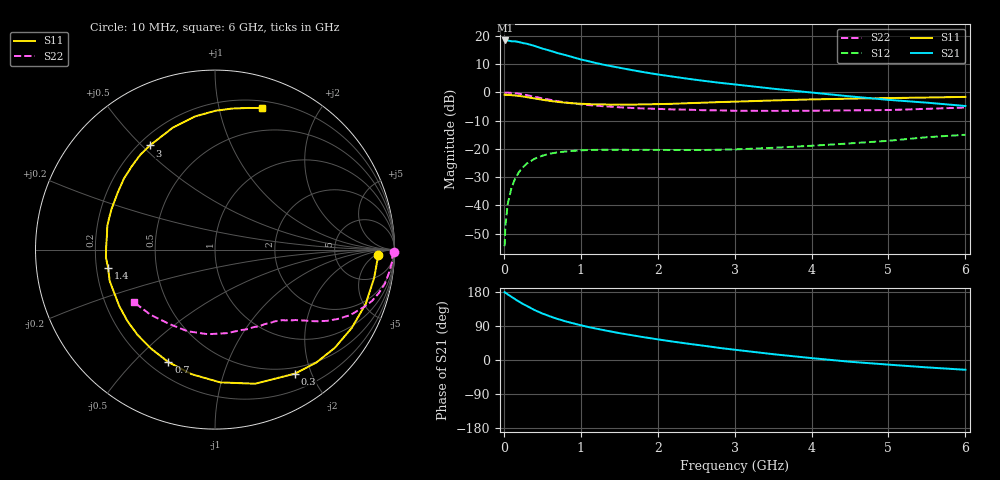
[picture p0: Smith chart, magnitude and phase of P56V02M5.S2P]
! SIEMENS Small Signal Semiconductors
! BFP183
! Si NPN RF Bipolar Junction Transistor in SOT143
! VCE = 6 V  IC = 2.5 mA
! Common Emitter S-Parameters:  March  1996
# GHz  S  MA  R  50
!  f  S11  S21  S12  S22
! GHz  MAG  ANG  MAG  ANG  MAG  ANG  MAG  ANG
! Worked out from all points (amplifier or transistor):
!   36 points, 10 MHz to 6 GHz, reference 50 ohm
!   highest |S21| = 18.4 dB at 20 MHz (marker M1)
!   |S21| within 3 dB of that: start of sweep to 518.8 MHz
!   unconditionally stable (mu >= 1): 2.027 GHz to 5.842 GHz
!   at 250 MHz: K = 0.13, MSG = 21.9 dB, |S12| = -26.4 dB
!   at 1.4 GHz: K = 0.71, MSG = 14.8 dB, |S12| = -20.3 dB
!   at 6 GHz: K = 0.97, MSG = 5.1 dB, |S12| = -15.0 dB
!   S11 on the Smith chart (normalised r, x): 10 MHz: 19, -6; 300 MHz: 0.41, -1.76; 700 MHz: 0.27, -0.63; 1.4 GHz: 0.25, -0.08; 3 GHz: 0.24, +0.53; 6 GHz: 0.26, +1.35
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0.01  0.9105 -1.8  8.196 178.8  0.0019 86.3  0.9971 -0.8
0.02  0.9056 -4.2  8.283 177.7  0.0043 90.3  0.9879 -1.5
0.05  0.9007 -10.1  8.274 173.3  0.0105 86.5  0.9894 -3.8
0.1  0.8927 -19.7  8.012 166.7  0.0206 78.4  0.9778 -7.7
0.15  0.8781 -29.8  7.97 160.1  0.0305 73.4  0.9645 -11.5
0.2  0.8631 -39.4  7.742 153.7  0.0394 68.3  0.9441 -14.9
0.3  0.8225 -57.1  7.24 142.5  0.0552 59.2  0.8914 -20.9
0.4  0.7801 -73.3  6.631 131.7  0.0669 51.3  0.8364 -25.9
0.5  0.7405 -87.7  5.961 122.8  0.0757 44.5  0.7837 -29.6
0.6  0.7063 -100.7  5.462 115.2  0.0824 39.2  0.7389 -32.5
0.7  0.6784 -112.5  4.948 108.3  0.0868 34.7  0.6981 -34.9
0.8  0.6567 -122.8  4.566 102.1  0.09 31.0  0.6647 -36.8
0.9  0.6417 -132.4  4.178 96.9  0.0923 27.8  0.6361 -38.4
1.1  0.6192 -149.5  3.56 86.9  0.0954 23.2  0.5955 -41.2
1.4  0.6041 -170.1  2.896 74.9  0.0968 18.4  0.557 -45.1
1.8  0.6142 167.7  2.3 60.8  0.0963 16.0  0.5197 -50.3
2.2  0.6279 149.8  1.896 48.5  0.0955 15.5  0.4987 -56.4
3  0.6844 122.0  1.382 27.1  0.0978 19.0  0.4726 -71.3
3.5  0.7188 109.1  1.161 15.4  0.1044 21.9  0.4701 -82.0
4.5  0.7737 89.8  0.849 -4.6  0.1251 24.7  0.4799 -108.7
5.5  0.8106 76.8  0.657 -19.5  0.1609 23.8  0.511 -134.8
6  0.8313 71.6  0.574 -25.8  0.1777 20.4  0.539 -147.2
